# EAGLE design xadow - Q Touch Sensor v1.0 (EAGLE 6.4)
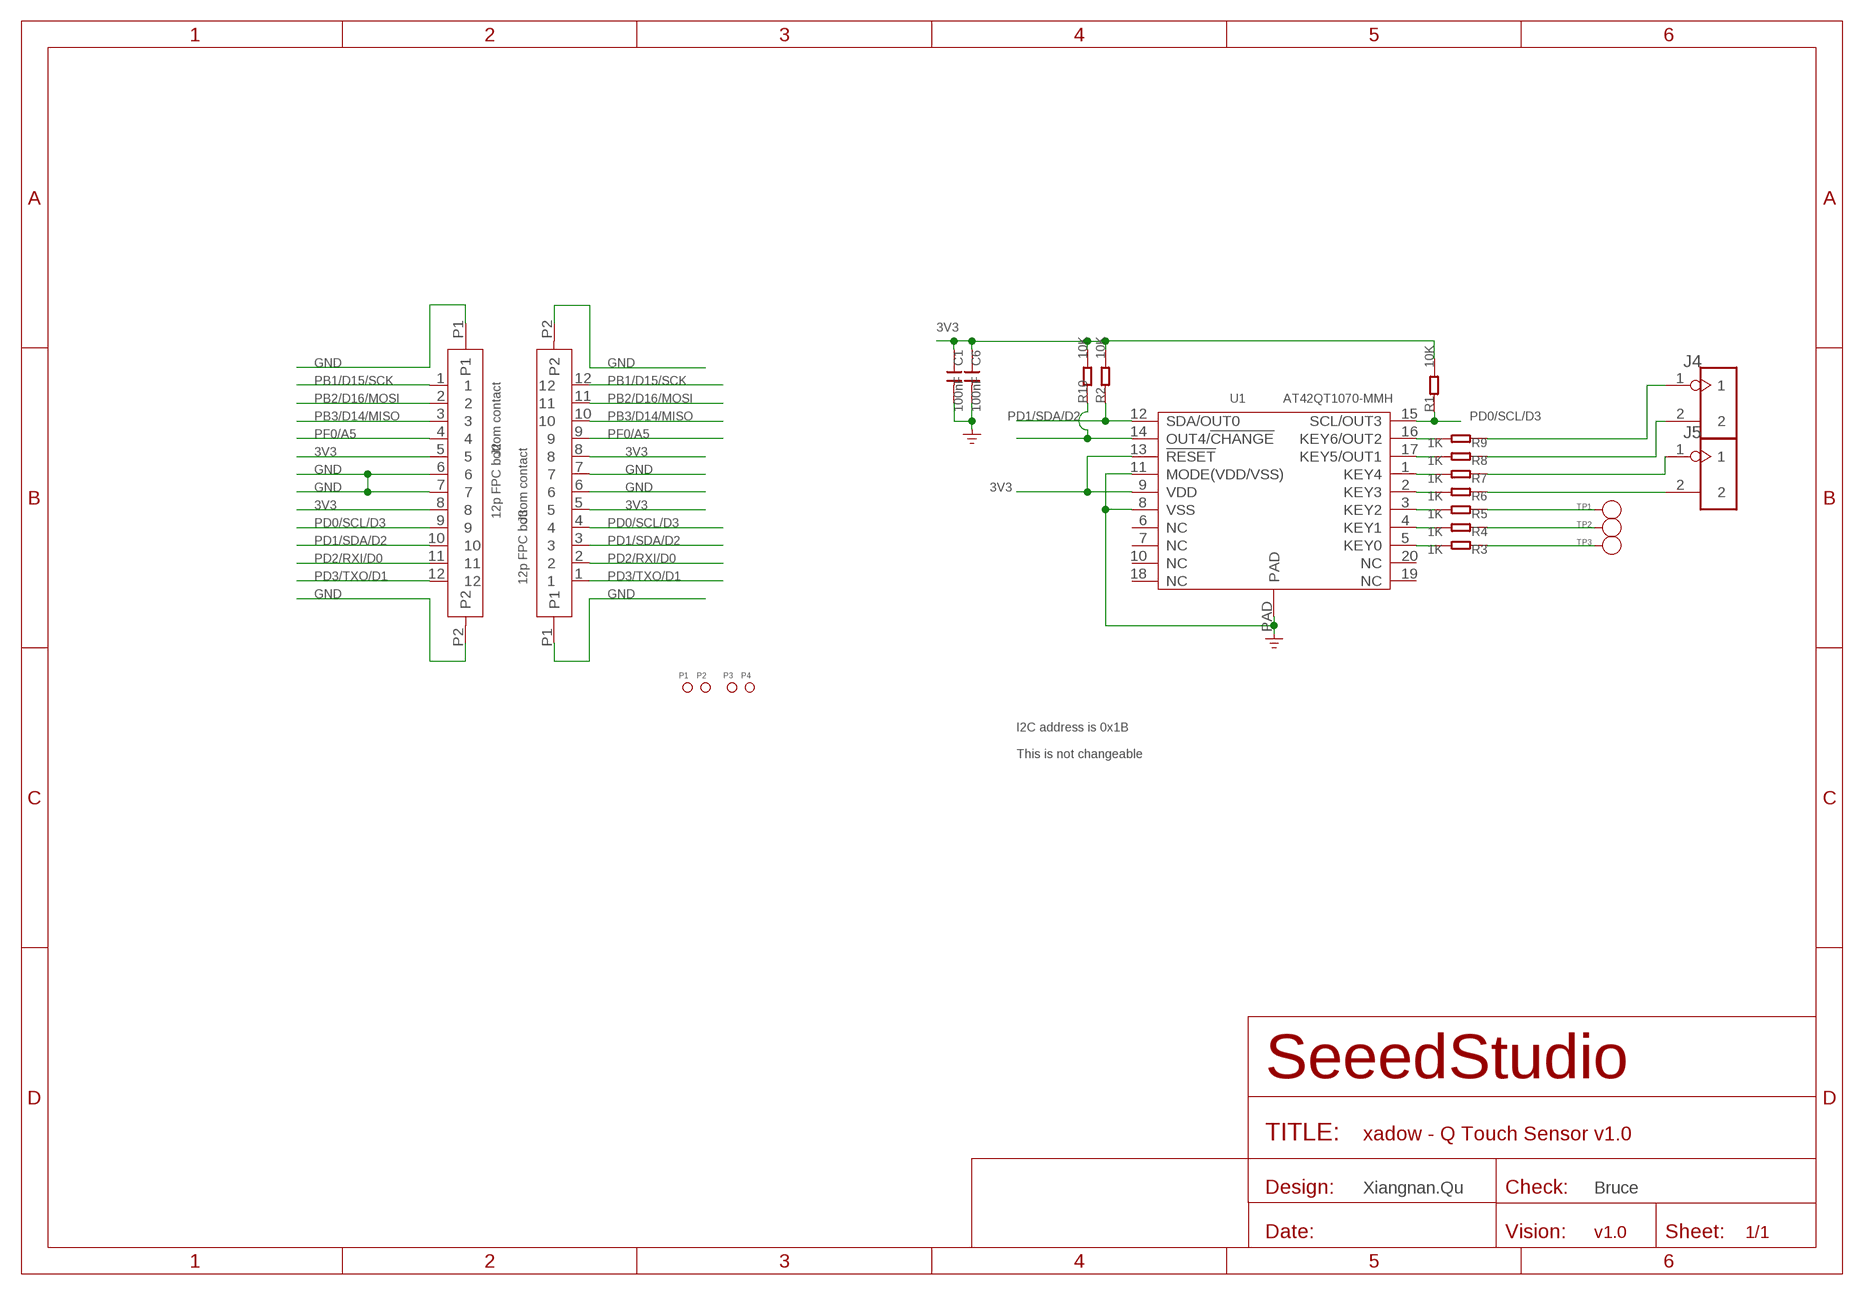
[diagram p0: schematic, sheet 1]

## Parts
C1  100nF  C-0402  [C0402]
C6  100nF  C-0402  [C0402]
J2  12p FPC bottom contact  FPC052002-12LT-FH12-12S-0.5SH  [12P-0.5-NEW]
J3  12p FPC bottom contact  FPC052002-12LT-FH12-12S-0.5SH  [12P-0.5-NEW]
J4  HEADER-2P-2.0  [2P-2.0]
J5  HEADER-2P-2.0  [2P-2.0]
P1  PAD-MARK  [ROUND-MARK-1.0]
P2  PAD-MARK  [ROUND-MARK-1.0]
P3  PAD-MARK  [ROUND-MARK-1.0]
P4  PAD-MARK  [ROUND-MARK-1.0]
R1  10K  R-0402  [R0402]
R2  10K  R-0402  [R0402]
R3  1K  R-0402  [R0402]
R4  1K  R-0402  [R0402]
R5  1K  R-0402  [R0402]
R6  1K  R-0402  [R0402]
R7  1K  R-0402  [R0402]
R8  1K  R-0402  [R0402]
R9  1K  R-0402  [R0402]
R10  10K  R-0402  [R0402]
TP1  PAD-TEST-POINT  [1P-D6MM]
TP2  PAD-TEST-POINT  [1P-D6MM]
TP3  PAD-TEST-POINT  [1P-D6MM]
U1  AT42QT1070-MMH  AT42QT1070MMH  [VQFN20-3X3]

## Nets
3V3: C1.1 C6.1 J2.5 J2.8 J3.5 J3.8 R1.2 R2.2 R10.2 U1.9(VDD) U1.13(!RESET)
GND: C1.2 C6.2 J2.6 J2.7 J2.P1 J2.P2 J3.6 J3.7 J3.P1 J3.P2 U1.8(VSS) U1.11(MODE(VDD/VSS)) U1.PAD
N$1: R9.2 U1.16(KEY6/OUT2)
N$2: R10.1 U1.14(OUT4/!CHANGE)
N$3: R8.2 U1.17(KEY5/OUT1)
N$5: J4.1 R9.1
N$6: J4.2 R8.1
N$7: R3.2 U1.5(KEY0)
N$8: R4.2 U1.4(KEY1)
N$9: R5.2 U1.3(KEY2)
N$10: R6.2 U1.2(KEY3)
N$11: R7.2 U1.1(KEY4)
N$20: J5.1 R7.1
N$21: J5.2 R6.1
N$22: R5.1 TP1.1(T)
N$23: R4.1 TP2.1(T)
N$24: R3.1 TP3.1(T)
PB1/D15/SCK: J2.1 J3.12
PB2/D16/MOSI: J2.2 J3.11
PB3/D14/MISO: J2.3 J3.10
PD0/SCL/D3: J2.9 J3.4 R1.1 U1.15(SCL/OUT3)
PD1/SDA/D2: J2.10 J3.3 R2.1 U1.12(SDA/OUT0)
PD2/RXI/D0: J2.11 J3.2
PD3/TXO/D1: J2.12 J3.1
PF0/A5: J2.4 J3.9
Unconnected: U1.6(NC) U1.7(NC) U1.10(NC) U1.18(NC) U1.19(NC) U1.20(NC)

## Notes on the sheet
- I2C address is 0x1B
- This is not changeable
- Xiangnan.Qu | Bruce
- v1.0

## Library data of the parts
C1 C6 = Discrete:C*: Ceramic Capacitors
J2 J3 = template :FPC052002-12LT
J4 J5 = Connector :HEADER-2P
P1-P4 = Discrete:PAD-MARK; PARTNO: DNP
R1-R10 = Discrete:R*
TP1-TP3 = Discrete:PAD-TEST-POINT
U1 = template :AT42QT1070MMH: Seven-channel QTouch® Touch Sensor IC

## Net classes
0 default: width 0.152 mm, drill 0.152 mm, clearance 0.152 mm

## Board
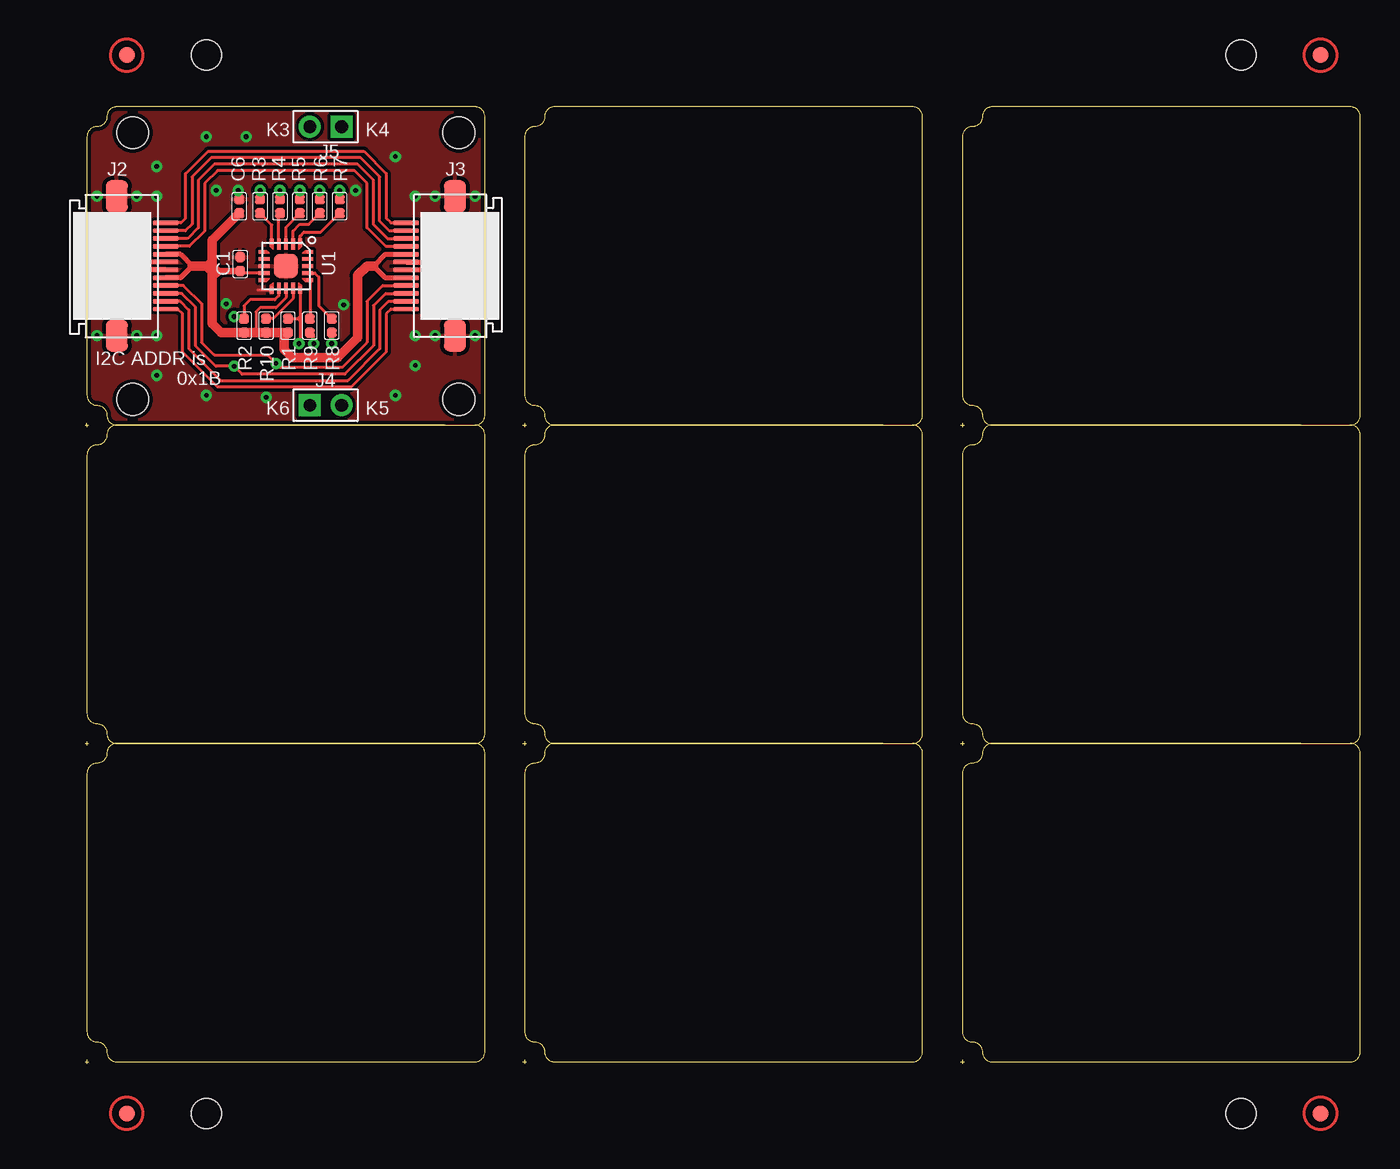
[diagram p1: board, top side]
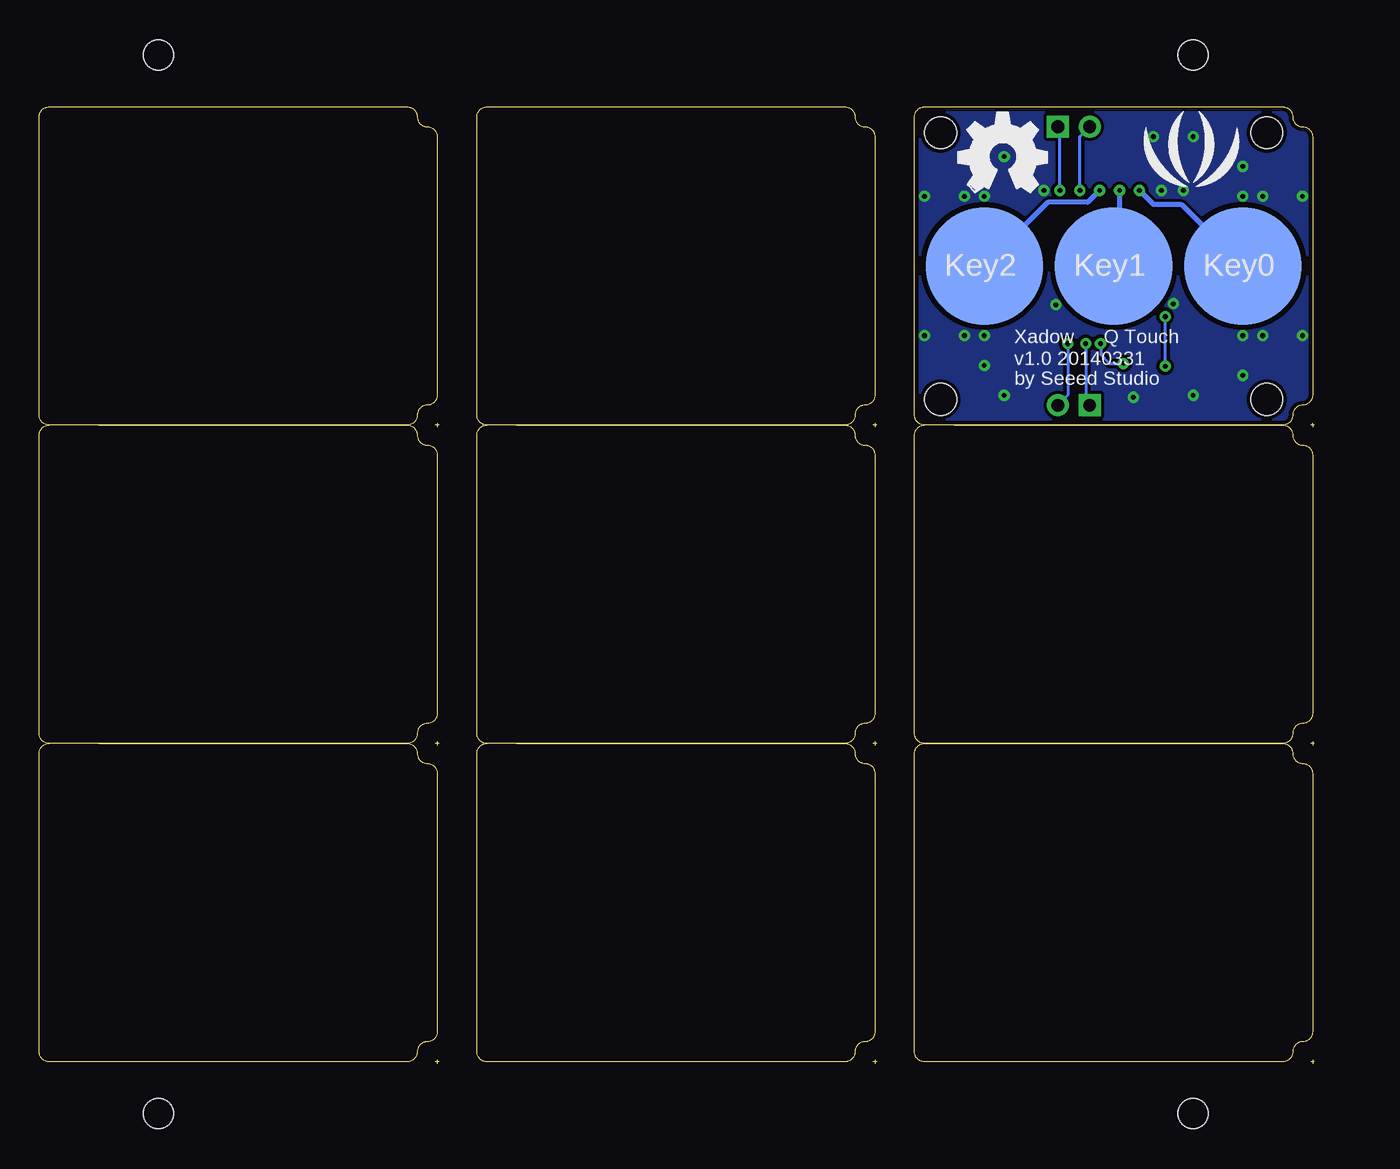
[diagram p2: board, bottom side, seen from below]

Size 81.41 x 61.09 mm. Coordinates in mm from the lower left corner, seen from the top.
Outline: 217 segments
Copper layers (1*16): Top 0.035mm / dielectric 1.5mm / Bottom 0.035mm
Design rules "default *": minimum track width 8mil, minimum drill 12mil, track to track 6mil, track to pad 6mil, pad to pad 6mil, via to via 6mil, smd to smd 0mil, copper to edge 10mil, drill to drill 8mil, minimum pad ring 10mil, minimum via ring 8mil, stop-mask expansion 4mil, vias tented up to drill 25mil, thermal gap 10mil
Holes 2.03 mm at 3.05,42.42 3.05,59.44 23.88,59.44 23.88,42.42
Holes 1.91 mm at 73.79,64.39 7.75,64.39 7.75,-3.17 73.79,-3.17
tRestrict: area 4.6,50.9 to 5.2,51; area 20.4,50.9 to 21,51; 13 lines
bRestrict: 13 lines

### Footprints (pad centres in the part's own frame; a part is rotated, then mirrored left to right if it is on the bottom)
C0402 = smd 0.635 x 0.635: 1 -0.445,0; 2 0.445,0
12P-0.5-NEW = smd 0.3 x 1.6: 1 -2.75,3.127; 2 -2.25,3.127; 3 -1.75,3.127; 4 -1.25,3.127; 5 -0.75,3.127; 6 -0.25,3.127; 7 0.25,3.127; 8 0.75,3.127; 9 1.25,3.127; 10 1.75,3.127; 11 2.25,3.127; 12 2.75,3.127 | smd 2.032 x 1.397: P1 -4.445,0; P2 4.445,0
2P-2.0 = drill 0.813 pad 1.397 square: 1 -1.016,0 | drill 0.813 pad 1.397: 2 1.016,0
ROUND-MARK-1.0 = smd 1.016 x 1.016: P$1 0,0
R0402 = smd 0.635 x 0.635: 1 -0.445,0; 2 0.445,0
1P-D6MM = smd 7.5 x 7.5: 1 0,0
VQFN20-3X3 = smd 0.4 x 0.25: 1 -1.55,0.9; 5 -1.55,-0.9; 11 1.55,-0.9; 15 1.55,0.9 | smd 0.7 x 0.25: 2 -1.4,0.45; 3 -1.4,0; 4 -1.4,-0.45; 12 1.4,-0.45; 13 1.4,0; 14 1.4,0.45 | smd 0.25 x 0.4: 6 -0.9,-1.55; 10 0.9,-1.55; 16 0.9,1.55; 20 -0.9,1.55 | smd 0.25 x 0.7: 7 -0.45,-1.4; 8 0,-1.4; 9 0.45,-1.4; 17 0.45,1.4; 18 0,1.4; 19 -0.45,1.4 | smd 1.55 x 1.55: PAD 0,0

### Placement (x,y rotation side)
C1  9.91,51.05 90 top
C6  9.84,54.74 90 top
J2  2.03,50.93 270 top
J3  23.62,50.93 90 top
J4  15.37,42.04 0 top
J5  15.37,59.82 180 top
P1  not placed on the board
P2  not placed on the board
P3  not placed on the board
P4  not placed on the board
R1  12.95,47.12 270 top
R2  10.16,47.12 270 top
R3  11.18,54.74 270 top
R4  12.45,54.74 270 top
R5  13.72,54.74 270 top
R6  14.99,54.74 270 top
R7  16.26,54.74 270 top
R8  15.75,47.12 90 top
R9  14.35,47.12 90 top
R10  11.56,47.12 270 top
TP1  21.08,50.93 180 bottom
TP2  12.83,50.93 180 bottom
TP3  4.57,50.93 180 bottom
U1  12.83,50.93 270 top
U$5  [LOGO_SILK]  7.87,57.66 0 bottom
U$6  [OSHW_FILLX200_NOTEXT]  22.73,55.63 0 bottom

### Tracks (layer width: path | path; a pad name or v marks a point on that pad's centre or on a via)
3V3
  Top 0.203: U1.9 9.84,50.48 9.91,50.55 C1.1 | U1.13 12.83,48.9 12.19,48.26 11.18,48.26 10.92,48.01 10.92,46.99 | 10.92,46.93 10.92,46.67 | 10.92,46.99 10.92,46.93 | 10.92,46.93 11.05,46.8 | 10.92,46.99 11.05,46.86 | 10.92,46.99 10.79,46.86
  Top 0.305: J2.5 6.11,51.68 6.86,50.93 6.11,50.18 J2.8 | J3.8 19.16,51.68 18.41,50.93 19.16,50.18 J3.5
  Top 0.406: C1.1 8.62,50.61 | 8.62,50.61 8.13,50.11 | 8.62,50.61 8.57,50.61 8.05,51.13
  Top 0.61: 18.41,50.93 18,50.93 17.4,50.33 17.4,46.36 16.13,45.09 13.21,45.09 12.7,45.59 12.7,46.67 | C6.1 8.13,52.58 8.13,51.24 | 12.7,46.67 R1.2 12.93,46.65 | 12.7,46.67 R10.2 10.92,46.67 R2.2 8.7,46.67 8.13,47.24 8.13,50.11 8.13,50.52 | 8.13,51.24 8.13,50.52 | 6.86,50.93 7.72,50.93 | 7.72,50.93 8.13,50.52 | 7.72,50.93 7.81,50.93 8.13,51.24
GND  (via drill 0.3 pad 0.64)
  Top 0.203: 21.84,50.67 21.84,50.68 22.1,50.68 22.22,50.68 22.22,50.67 | 3.81,50.67 3.81,50.68 3.17,50.68 1.15,50.68 | 3.81,51.18 3.43,51.18 1.14,51.18 | U1.11 11.05,49.38 11.05,49.4
  Top 0.305: J2.6 3.43,51.18 | J2.7 3.17,50.68 | J3.6 22.1,50.68 | J3.7 22.61,51.18 22.61,51.05
  other vias: 24.89,55.37 24.89,46.48 9.78,55.75 0.76,46.48 0.76,55.37 8.38,55.75 4.57,55.37 3.3,46.48 3.3,55.37 4.57,46.48 22.35,46.48 21.08,46.48 21.08,55.37 22.35,55.37 9.02,48.51 16.51,48.45 17.27,55.75 4.57,57.28 7.75,59.18 10.29,59.18 19.81,57.91 4.57,43.94 7.75,42.67 11.56,42.55 19.81,42.67 21.08,44.58
  pour Top (isolate 0.203): 25.53,61.09 0.13,61.09 0.13,40.77 25.53,40.77
  pour Bottom (isolate 0.203): 25.53,61.09 0.13,61.09 0.13,40.77 25.53,40.77
N$1
  Top 0.203: U1.16 14.38,47.59 R9.2
N$2
  Top 0.203: U1.14 13.28,48.84 12,47.56 R10.1
N$3
  Top 0.203: U1.17 14.67,50.48 14.92,50.23 14.92,48.39 R8.2
N$5  (via drill 0.3 pad 0.64)
  Top 0.203: v14.61,45.97 14.61,46.42 R9.1
  Bottom 0.203: v14.61,45.97 14.61,42.29 J4.1
N$6  (via drill 0.3 pad 0.64)
  Top 0.203: R8.1 v15.75,45.97
  Bottom 0.203: v15.75,45.97 15.75,42.67 J4.2
N$7
  Top 0.203: U1.5 11.93,53.54 R3.2
N$8
  Top 0.203: U1.4 12.38,54.16 12.45,54.23 R4.2
N$9
  Top 0.203: U1.3 12.83,53.4 R5.2
N$10
  Top 0.203: U1.2 13.28,53.16 13.72,53.59 14.29,53.59 R6.2
N$11
  Top 0.203: U1.1 13.73,52.84 13.97,53.09 15.05,53.09 R7.2
N$20  (via drill 0.3 pad 0.64)
  Top 0.203: R7.1 v16.26,55.75
  Bottom 0.203: v16.26,55.75 16.26,59.69 J5.1
N$21  (via drill 0.3 pad 0.64)
  Top 0.203: R6.1 v14.99,55.75
  Bottom 0.203: v14.99,55.75 14.99,59.18 J5.2
N$22  (via drill 0.3 pad 0.64)
  Top 0.203: R5.1 v13.72,55.75
  Bottom 0.305: v13.72,55.75 14.48,54.99 17.02,54.99 TP1.1
N$23  (via drill 0.3 pad 0.64)
  Top 0.305: R4.1 v12.45,55.75
  Bottom 0.305: v12.45,55.75 12.45,51.31 TP2.1
N$24  (via drill 0.3 pad 0.64)
  Top 0.305: R3.1 v11.18,55.75
  Bottom 0.305: v11.18,55.75 10.29,54.86 8.51,54.86 TP3.1
PB1/D15/SCK
  Top 0.203: J2.1 6.13,53.68 6.43,53.98 6.43,56.82 7.85,58.24 17.8,58.24 19.23,56.82 19.23,53.98 19.53,53.68 J3.12
PB2/D16/MOSI
  Top 0.203: J2.2 6.41,53.18 6.83,53.6 6.83,56.62 8.05,57.84 17.6,57.84 18.82,56.62 18.82,53.77 19.42,53.18 J3.11
PB3/D14/MISO
  Top 0.203: J2.3 6.55,52.68 7.24,53.37 7.24,56.41 8.26,57.43 17.4,57.43 18.41,56.41 18.41,53.57 19.31,52.68 J3.10
PD0/SCL/D3  (via drill 0.3 pad 0.64)
  Top 0.203: U1.15 13.73,47.62 | R1.1 13.59,47.56 | 13.59,47.56 13.66,47.56 13.73,47.62 | 13.73,47.62 13.73,46.05 v13.65,45.97 | 13.59,47.56 13.72,47.44 | 13.59,47.56 13.72,47.69 | J2.9 6.27,49.68 7.44,48.51 7.44,46.05 8.26,45.24 11.66,45.24 v12.19,44.7 12.45,44.45 16.41,44.45 18.01,46.05 18.01,48.68 19.01,49.68 J3.4
  Bottom 0.203: v13.65,45.97 13.65,45.28 13.08,44.7 v12.19,44.7
PD1/SDA/D2  (via drill 0.3 pad 0.64)
  Top 0.203: U1.12 12.38,49.03 12.11,48.77 10.54,48.77 10.16,48.39 R2.1 9.67,47.56 v9.53,47.7 | J2.10 6.17,49.18 7.04,48.32 7.04,45.85 8.36,44.53 v9.53,44.53 9.53,44.51 10.02,44.02 16.59,44.02 18.41,45.85 18.41,48.4 19.19,49.18 J3.3
  Bottom 0.203: v9.53,44.53 v9.53,47.7
PD2/RXI/D0
  Top 0.203: J2.11 6.06,48.68 6.63,48.11 6.63,45.64 8.66,43.61 16.79,43.61 18.82,45.64 18.82,48.11 19.39,48.68 J3.2
PD3/TXO/D1
  Top 0.203: J2.12 5.92,48.18 6.22,47.88 6.22,45.44 8.46,43.21 16.99,43.21 19.23,45.44 19.23,47.88 19.53,48.18 J3.1
PF0/A5
  Top 0.203: J2.4 6.66,52.18 7.64,53.16 7.64,56.21 8.46,57.02 17.2,57.02 18.01,56.21 18.01,53.37 19.2,52.18 J3.9

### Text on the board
tPlace: K3 | K4 | I2C ADDR is | 0x1B | K6 | K5
bPlace: Key0 | Key1 | Key2 | Q Touch | Xadow | v1.0 20140331 | by Seeed Studio
Patch_Top: Top Enhance 0.25~0.28mm
Vscore: Bottom Enhance
tMap: Holes on Bottom Enhance | All Holes are 70mil diameter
